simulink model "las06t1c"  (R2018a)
settings: Solver=ode45  StartTime=0.0  StopTime=10  MaxStep=10  MinStep=0.0001  RelTol=1e-3  AbsTol=1e-3  EnableMultiTasking=on
libraries: simulink x1

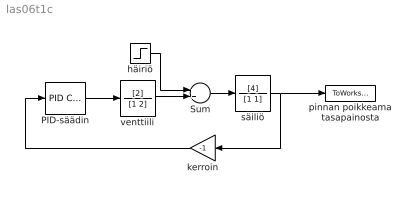
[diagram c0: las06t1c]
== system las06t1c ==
  PID-säädin : simulink/Continuous/PID Controller  Controller=PID  TimeDomain=Continuous-time  SampleTime=-1  IntegratorMethod=Forward Euler  FilterMethod=Forward Euler  Form=Parallel  UseFilter=on  ControllerParametersSource=internal  P=2  I=1  D=0  N=100  InitialConditionSource=internal  InitialConditionForIntegrator=0  InitialConditionForFilter=0  ExternalReset=none  LimitOutput=off  UpperSaturationLimit=inf  LowerSaturationLimit=-inf  LinearizeAsGain=on  AntiWindupMode=none  Kb=1  TrackingMode=off  Kt=1  PParamMin=[]  PParamMax=[]  IParamMin=[]  IParamMax=[]  DParamMin=[]  DParamMax=[]  NParamMin=[]  NParamMax=[]  KbParamMin=[]  KbParamMax=[]  KtParamMin=[]  KtParamMax=[]  POutMin=[]  POutMax=[]  IOutMin=[]  IOutMax=[]  DOutMin=[]  DOutMax=[]  NOutMin=[]  NOutMax=[]  KbOutMin=[]  KbOutMax=[]  KtOutMin=[]  KtOutMax=[]  IntegratorOutMin=[]  IntegratorOutMax=[]  FilterOutMin=[]  FilterOutMax=[]  SumOutMin=[]  SumOutMax=[]  SumI1OutMin=[]  SumI1OutMax=[]  SumI2OutMin=[]  SumI2OutMax=[]  SumI3OutMin=[]  SumI3OutMax=[]  SumDOutMin=[]  SumDOutMax=[]  SaturationOutMin=[]  SaturationOutMax=[]  IntegratorContinuousStateAttributes=''  IntegratorStateMustResolveToSignalObject=off  IntegratorRTWStateStorageClass=Auto  FilterContinuousStateAttributes=''  FilterStateMustResolveToSignalObject=off  FilterRTWStateStorageClass=Auto  DifferentiatorICPrevScaledInput=0  DifferentiatorOutMin=[]  DifferentiatorOutMax=[]  FilterDiffOutCoefMin=[]  FilterDiffOutCoefMax=[]  SumDenOutMin=[]  SumDenOutMax=[]  SumNumOutMin=[]  SumNumOutMax=[]  ReciprocalOutMin=[]  ReciprocalOutMax=[]  DivideOutMin=[]  DivideOutMax=[]  TunerSelectOption=Transfer Function Based (PID Tuner App)
  Sum : Sum
  häiriö : Step  Time=3  After=-1
  kerroin : Gain  Gain=-1
  pinnan poikkeama tasapainosta : ToWorkspace  VariableName=y
  säiliö : TransferFcn  Numerator=[4]  Denominator=[1 1]
  venttiili : TransferFcn  Numerator=[2]  Denominator=[1 2]
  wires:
  häiriö/1 -> Sum/1
  venttiili/1 -> Sum/2
  Sum/1 -> säiliö/1
  säiliö/1 -> pinnan poikkeama tasapainosta/1, kerroin/1
  PID-säädin/1 -> venttiili/1
  kerroin/1 -> PID-säädin/1
